(* Logix 5000 AddOnInstructionDefinition export YAI_Assy_155_115_EIP_Hz; software revision 21.03 *)

ADD_ON_INSTRUCTION YAI_Assy_155_115_EIP_Hz   (* revision 1.0, vendor Yaskawa America, Inc. *)
// YAI Assembly 155 and 115
// Help:
// This add-on instruction is for use with input assemblie 166 and output assemblies 116.
// Node_Input_Assy is defined as the node's input assembly integer array.
// Node_Output_Assy is defined as the node's output assembly integer array.
// Torque limit/reference, torque compensation and torque output variables are only available with A1000.
VAR_IN_OUT
   Node_Input_Assy : AB:ETHERNET_MODULE_INT_40Bytes:I:0; {required}   // Input assembly words
   Node_Output_Assy : AB:ETHERNET_MODULE_INT_40Bytes:O:0; {required}   // Output assembly words
END_VAR
VAR_INPUT
   RunFwd : BOOL; {visible}   // Forward run command
   RunRev : BOOL; {visible}   // Reverse run command
   MFI_3 : BOOL; {visible}   // Multi-function input 3
   MFI_4 : BOOL; {visible}   // Multi-function input 4
   MFI_5 : BOOL; {visible}   // Multi-function input 5
   MFI_6 : BOOL; {visible}   // Multi-function input 6
   MFI_7 : BOOL; {visible}   // Multi-function input 7
   MFI_8 : BOOL; {visible}   // Multi-function input 8
   External_Fault : BOOL;   // External fault command (EF0)
   FaultReset : BOOL; {visible}   // Fault reset command
   MFO_1 : BOOL; {visible}   // Multi-function output (M1-M2 for A/P1000, MA/MB/MC for V1000)
   MFO_2 : BOOL; {visible}   // Multi-function output (M3-M4 for A/P1000, P1 for V1000)
   MFO_3 : BOOL; {visible}   // Multi-function output (M5-M6 for A/P1000, P2 for V1000)
   Freq_Ref : REAL; {visible}   // Frequency reference command in Hz (xx.xx resolution)
   Torq_Ref_Limit : REAL; {visible}   // Torque reference/limit (A1000 only)
   Torq_Comp : REAL; {visible}   // Torque compensation command (A1000 only)
   Analog_Output_1 : REAL;   // Analog output 1 level command
   Analog_Output_2 : REAL;   // Analog output 2 level command
   Digital_Output_1 : BOOL;   // Digital output 1 activation - M1-M2
   Digital_Output_2 : BOOL;   // Digital output 2 activation - M3-M4
   Digital_Output_3 : BOOL;   // Digital output 3 activation - M5-M6
   Digital_Output_Fault_Enable : BOOL;   // Bit to enable control of fault output relay over the network
   Digital_Output_Fault : BOOL;   // Fault relay activation - MA-MB-MC
END_VAR
VAR_OUTPUT
   Running : BOOL; {access Read Only, visible}   // Drive running forward status bit
   ZSP : BOOL; {access Read Only, visible}   // Drive zero speed status bit
   RunningRev : BOOL; {access Read Only, visible}   // Drive running reverse status bit
   Reset : BOOL; {access Read Only, visible}   // Drive reset command status bit
   At_Speed : BOOL; {access Read Only, visible}   // Drive at commanded speed status bit
   Ready : BOOL; {access Read Only, visible}   // Drive ready status bit
   Alarm : BOOL; {access Read Only, visible}   // Drive alarm status bit
   Faulted : BOOL; {access Read Only, visible}   // Drive faulted status bit
   OPE : BOOL; {access Read Only}   // OPE alarm/fault present
   UV : BOOL; {access Read Only}   // Drive in UV (undervoltage) state status bit
   NetCtrlStatus : BOOL; {access Read Only, visible}   // Drive network run source status bit (1 = source coming from network)
   MFO_1_Status : BOOL; {access Read Only, visible}   // Drive multi-function output 1 (M1-M2 for A/P1000, MA/MB/MC for V1000) status
   MFO_2_Status : BOOL; {access Read Only, visible}   // Drive multi-function output 1 (M3-M4 for A/P1000, P1 for V1000) status
   MFO_3_Status : BOOL; {access Read Only, visible}   // Drive multi-function output 1 (M5-M6 for A/P1000, P2 for V1000) status
   ZSV : BOOL; {access Read Only, visible}   // Drive zero servo completed status bit
   Motor_Speed : REAL; {access Read Only, visible}   // Motor speed in Hz (xx.xx resolution)
   Torque_Actual : REAL; {access Read Only, visible}   // Drive torque output in % (xxx.x resolution)
   PG1_Count : INT; {access Read Only}   // Encoder feedback count
   Freq_Cmd : REAL; {access Read Only, visible}   // Commanded frequency in Hz (xx.xx resolution)
   Output_Freq : REAL; {access Read Only, visible}   // Drive output frequency in Hz (xx.xx resolution)
   Output_Current : REAL; {access Read Only, visible}   // Drive output current in A (xxx.x resolution)
   Analog_Input_1_Level : REAL; {access Read Only}   // Analog input 1 level in % (xxx.x resolution)
   DC_Bus_Volt : INT; {access Read Only, visible}   // DC bus voltage in Vdc (xxx resolution)
   Analog_Input_3_Level : REAL; {access Read Only}   // Analog input 3 level in % (xxx.x resolution)
   Analog_Input_2_Level : REAL; {access Read Only}   // Analog input 2 level in % (xxx.x resolution)
   S1_Status : BOOL; {access Read Only}   // Digital input S1 status
   S2_Status : BOOL; {access Read Only}   // Digital input S2 status
   S3_Status : BOOL; {access Read Only}   // Digital input S3 status
   S4_Status : BOOL; {access Read Only}   // Digital input S4 status
   S5_Status : BOOL; {access Read Only}   // Digital input S5 status
   S6_Status : BOOL; {access Read Only}   // Digital input S6 status
   S7_Status : BOOL; {access Read Only}   // Digital input S7 status
   S8_Status : BOOL; {access Read Only}   // Digital input S8 status
   PG2_Count : INT;   // Encoder 2 feedback count
   UV_Alarm : BOOL; {access Read Only}   // Undervoltage alarm
   OV_Alarm : BOOL; {access Read Only}   // Overvoltage alarm
   OH_Alarm : BOOL; {access Read Only}   // Overheat alarm
   OH2_Alarm : BOOL; {access Read Only}   // Drive overheat alarm
   OL3_Alarm : BOOL; {access Read Only}   // Overtorque detection 1 alarm
   OL4_Alarm : BOOL; {access Read Only}   // Overtorque detection 2 alarm
   EF_Alarm : BOOL; {access Read Only}   // Run command error alarm
   bb_Alarm : BOOL; {access Read Only}   // Baseblock alarm
   EF3_Alarm : BOOL; {access Read Only}   // External fault 3 alarm
   EF4_Alarm : BOOL; {access Read Only}   // External fault 4 alarm
   EF5_Alarm : BOOL; {access Read Only}   // External fault 5 alarm
   EF6_Alarm : BOOL; {access Read Only}   // External fault 6 alarm
   EF7_Alarm : BOOL; {access Read Only}   // External fault 7 alarm
   EF8_Alarm : BOOL; {access Read Only}   // External fault 8 alarm
   FAN_Alarm : BOOL; {access Read Only}   // Cooling fan error alarm
   OS_Alarm : BOOL; {access Read Only}   // Overspeed alarm
   DEV_Alarm : BOOL; {access Read Only}   // Speed deviation alarm
   PGO_Alarm : BOOL; {access Read Only}   // Encoder feedback open alarm
   OPR_Alarm : BOOL; {access Read Only}   // Operator removed alarm
   CE_Alarm : BOOL; {access Read Only}   // Serial communication error alarm
   BUS_Alarm : BOOL; {access Read Only}   // BUS alarm
   CALL_Alarm : BOOL; {access Read Only}   // Serial communication timeout alarm
   OL1_Alarm : BOOL; {access Read Only}   // Motor overload alarm
   OL2_Alarm : BOOL; {access Read Only}   // Drive overload alarm
   EF0_Alarm : BOOL; {access Read Only}   // External fault 0 alarm
   RUN_Alarm : BOOL; {access Read Only}   // Motor 2 run command issued while running alarm
   UL3_Alarm : BOOL; {access Read Only}   // Undertorque detecxtion 1 alarm
   UL4_Alarm : BOOL; {access Read Only}   // Undertorque detection 2 alarm
   SE_Alarm : BOOL; {access Read Only}   // Modbus test failure alarm
   OH3_Alarm : BOOL; {access Read Only}   // Motor overload alarm
   FBL_Alarm : BOOL; {access Read Only}   // PID feedback loss alarm
   FBH_Alarm : BOOL; {access Read Only}   // PID feedback loss alarm
   DNE_Alarm : BOOL; {access Read Only}   // Drive not enabled alarm
END_VAR
VAR
   FRef_Convert : DINT;
   FOut_Convert : REAL;
   FOut_Temp : REAL;
   TRef_Convert : INT;
   TComp_Convert : INT;
   TOut_Convert : REAL;
   TOut_Temp : REAL;
   IOut_Temp : REAL;
   IOut_Convert : REAL;
   AO1_Convert : INT;
   AO2_Convert : INT;
   Motor_Speed_Temp : REAL;
   Motor_Speed_Convert : REAL;
   Freq_Cmd_Temp : REAL;
   Freq_Cmd_Convert : REAL;
   AI1_Temp : REAL;
   AI1_Convert : REAL;
   AI2_Temp : REAL; {access None}
   AI2_Convert : REAL; {access None}
   AI3_Temp : REAL; {access None}
   AI3_Convert : REAL; {access None}
END_VAR

ROUTINE Logic   (* ladder *)
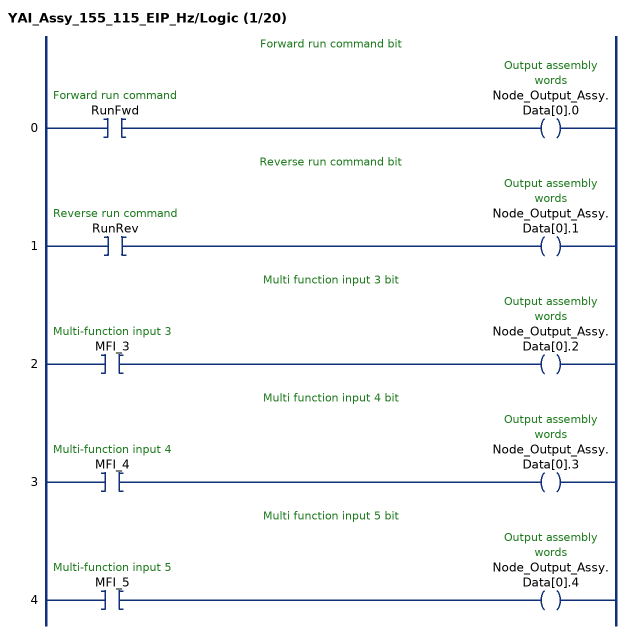
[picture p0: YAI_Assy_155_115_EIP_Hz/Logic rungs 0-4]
   // Forward run command bit
   0: XIC(RunFwd)OTE(Node_Output_Assy.Data[0].0);
   // Reverse run command bit
   1: XIC(RunRev)OTE(Node_Output_Assy.Data[0].1);
   // Multi function input 3 bit
   2: XIC(MFI_3)OTE(Node_Output_Assy.Data[0].2);
   // Multi function input 4 bit
   3: XIC(MFI_4)OTE(Node_Output_Assy.Data[0].3);
   // Multi function input 5 bit
   4: XIC(MFI_5)OTE(Node_Output_Assy.Data[0].4);
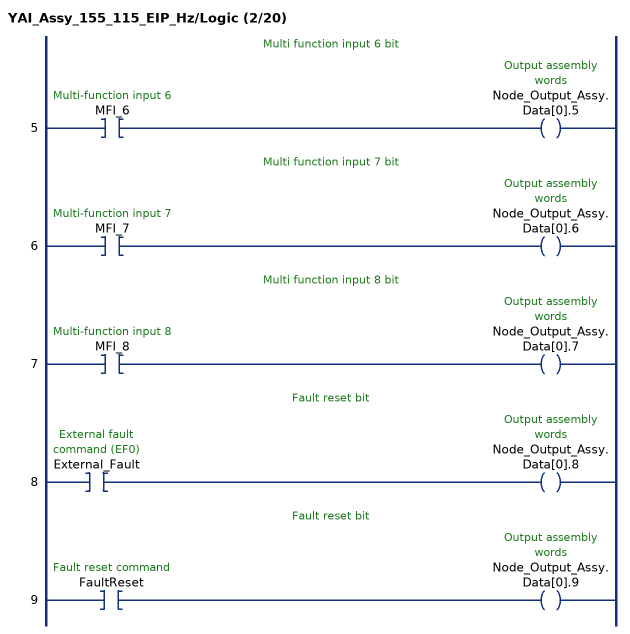
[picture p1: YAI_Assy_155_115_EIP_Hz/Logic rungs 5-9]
   // Multi function input 6 bit
   5: XIC(MFI_6)OTE(Node_Output_Assy.Data[0].5);
   // Multi function input 7 bit
   6: XIC(MFI_7)OTE(Node_Output_Assy.Data[0].6);
   // Multi function input 8 bit
   7: XIC(MFI_8)OTE(Node_Output_Assy.Data[0].7);
   // Fault reset bit
   8: XIC(External_Fault)OTE(Node_Output_Assy.Data[0].8);
   // Fault reset bit
   9: XIC(FaultReset)OTE(Node_Output_Assy.Data[0].9);
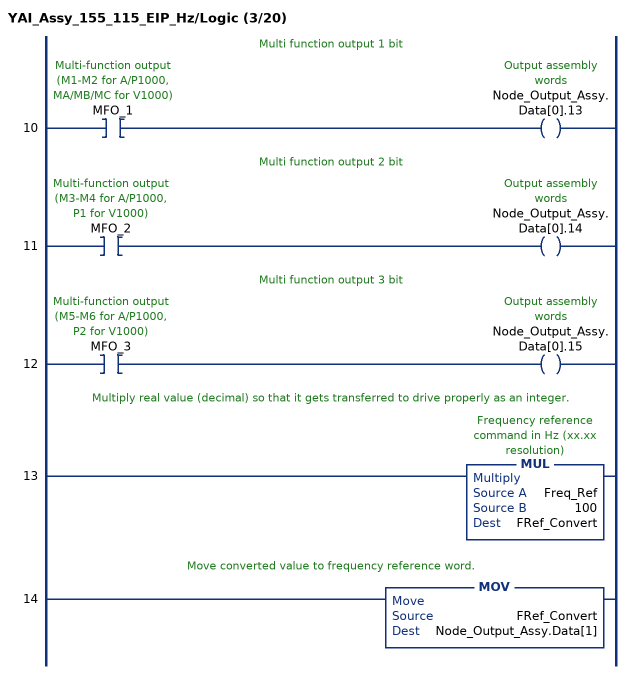
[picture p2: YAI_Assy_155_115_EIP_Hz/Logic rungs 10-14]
   // Multi function output 1 bit
   10: XIC(MFO_1)OTE(Node_Output_Assy.Data[0].13);
   // Multi function output 2 bit
   11: XIC(MFO_2)OTE(Node_Output_Assy.Data[0].14);
   // Multi function output 3 bit
   12: XIC(MFO_3)OTE(Node_Output_Assy.Data[0].15);
   // Multiply real value (decimal) so that it gets transferred to drive properly as an integer.
   13: MUL(Freq_Ref,100,FRef_Convert);
   // Move converted value to frequency reference word.
   14: MOV(FRef_Convert,Node_Output_Assy.Data[1]);
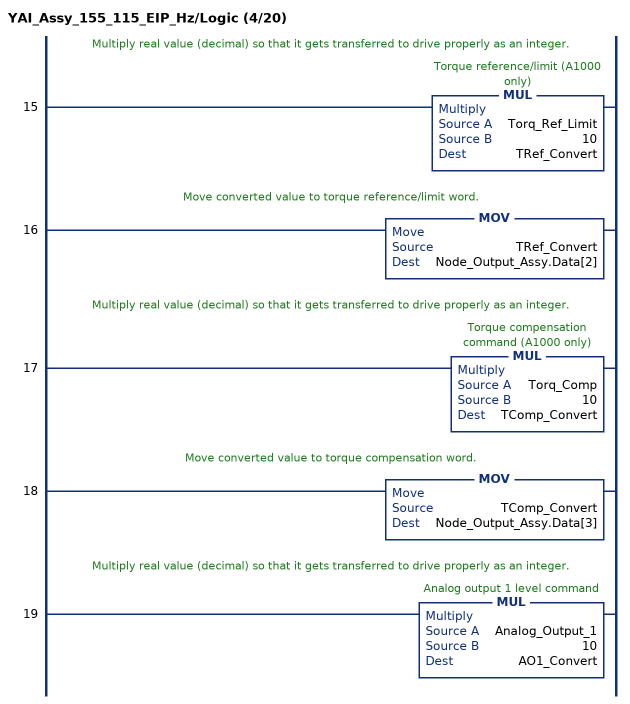
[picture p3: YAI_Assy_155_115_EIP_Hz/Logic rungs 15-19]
   // Multiply real value (decimal) so that it gets transferred to drive properly as an integer.
   15: MUL(Torq_Ref_Limit,10,TRef_Convert);
   // Move converted value to torque reference/limit word.
   16: MOV(TRef_Convert,Node_Output_Assy.Data[2]);
   // Multiply real value (decimal) so that it gets transferred to drive properly as an integer.
   17: MUL(Torq_Comp,10,TComp_Convert);
   // Move converted value to torque compensation word.
   18: MOV(TComp_Convert,Node_Output_Assy.Data[3]);
   // Multiply real value (decimal) so that it gets transferred to drive properly as an integer.
   19: MUL(Analog_Output_1,10,AO1_Convert);
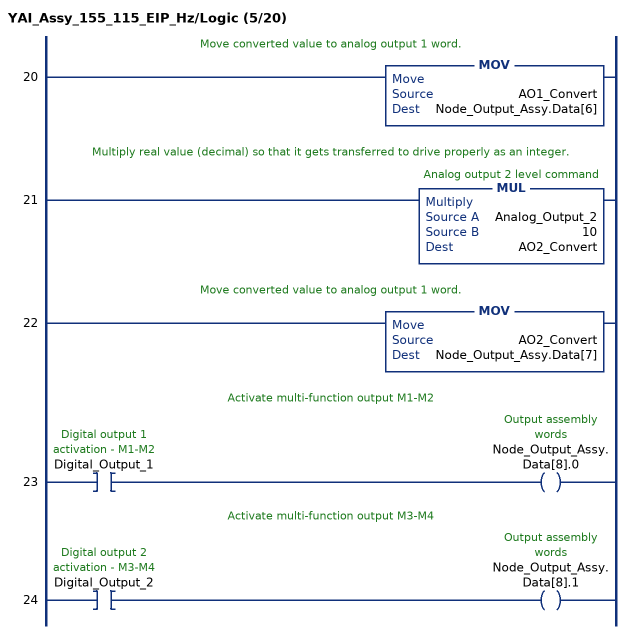
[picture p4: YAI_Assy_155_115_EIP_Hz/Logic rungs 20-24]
   // Move converted value to analog output 1 word.
   20: MOV(AO1_Convert,Node_Output_Assy.Data[6]);
   // Multiply real value (decimal) so that it gets transferred to drive properly as an integer.
   21: MUL(Analog_Output_2,10,AO2_Convert);
   // Move converted value to analog output 1 word.
   22: MOV(AO2_Convert,Node_Output_Assy.Data[7]);
   // Activate multi-function output M1-M2
   23: XIC(Digital_Output_1)OTE(Node_Output_Assy.Data[8].0);
   // Activate multi-function output M3-M4
   24: XIC(Digital_Output_2)OTE(Node_Output_Assy.Data[8].1);
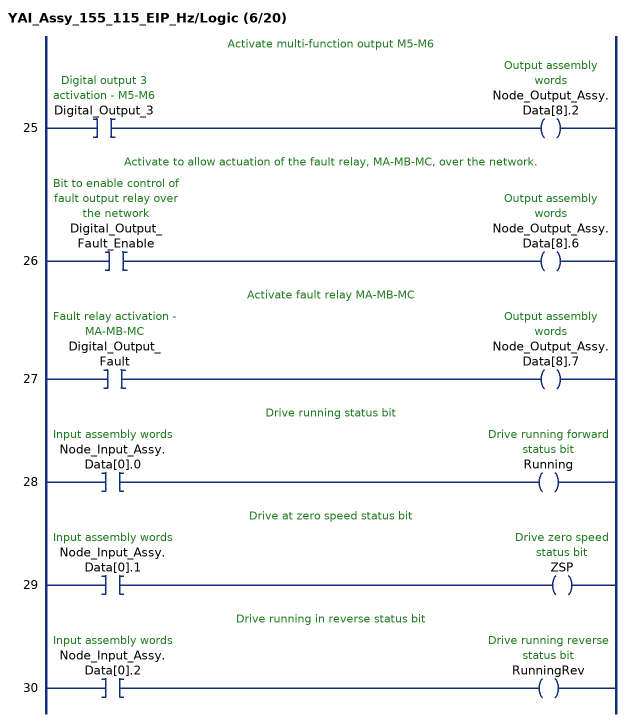
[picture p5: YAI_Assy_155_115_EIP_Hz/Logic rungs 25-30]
   // Activate multi-function output M5-M6
   25: XIC(Digital_Output_3)OTE(Node_Output_Assy.Data[8].2);
   // Activate to allow actuation of the fault relay, MA-MB-MC, over the network.
   26: XIC(Digital_Output_Fault_Enable)OTE(Node_Output_Assy.Data[8].6);
   // Activate fault relay MA-MB-MC
   27: XIC(Digital_Output_Fault)OTE(Node_Output_Assy.Data[8].7);
   // Drive running status bit
   28: XIC(Node_Input_Assy.Data[0].0)OTE(Running);
   // Drive at zero speed status bit
   29: XIC(Node_Input_Assy.Data[0].1)OTE(ZSP);
   // Drive running in reverse status bit
   30: XIC(Node_Input_Assy.Data[0].2)OTE(RunningRev);
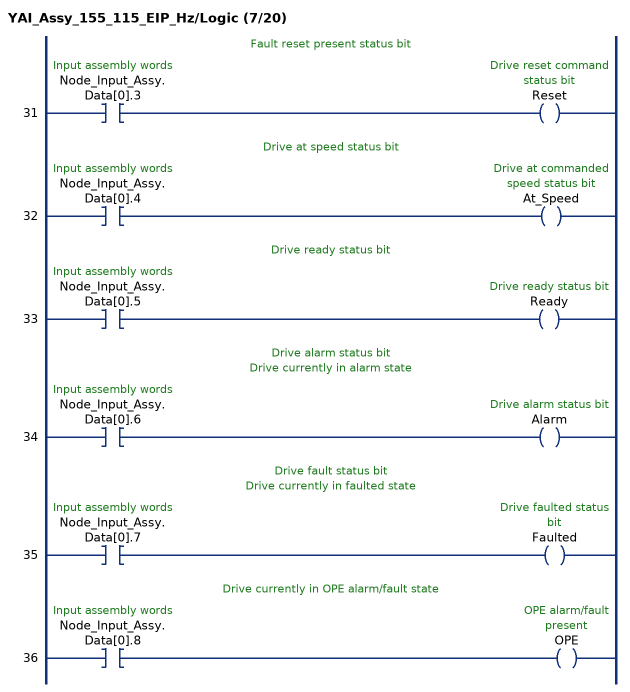
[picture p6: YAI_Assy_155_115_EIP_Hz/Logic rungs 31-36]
   // Fault reset present status bit
   31: XIC(Node_Input_Assy.Data[0].3)OTE(Reset);
   // Drive at speed status bit
   32: XIC(Node_Input_Assy.Data[0].4)OTE(At_Speed);
   // Drive ready status bit
   33: XIC(Node_Input_Assy.Data[0].5)OTE(Ready);
   // Drive alarm status bit
   // Drive currently in alarm state
   34: XIC(Node_Input_Assy.Data[0].6)OTE(Alarm);
   // Drive fault status bit
   // Drive currently in faulted state
   35: XIC(Node_Input_Assy.Data[0].7)OTE(Faulted);
   // Drive currently in OPE alarm/fault state
   36: XIC(Node_Input_Assy.Data[0].8)OTE(OPE);
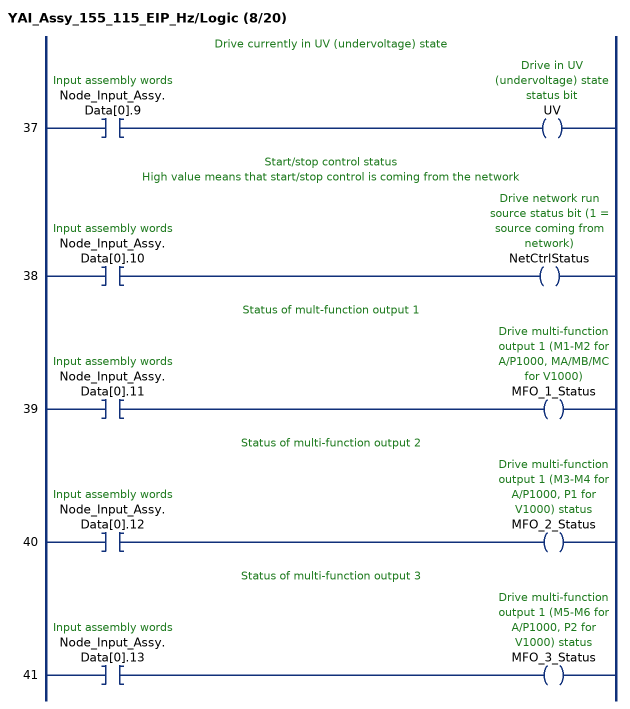
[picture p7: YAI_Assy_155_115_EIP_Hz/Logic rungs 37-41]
   // Drive currently in UV (undervoltage) state
   37: XIC(Node_Input_Assy.Data[0].9)OTE(UV);
   // Start/stop control status
   // High value means that start/stop control is coming from the network
   38: XIC(Node_Input_Assy.Data[0].10)OTE(NetCtrlStatus);
   // Status of mult-function output 1
   39: XIC(Node_Input_Assy.Data[0].11)OTE(MFO_1_Status);
   // Status of multi-function output 2
   40: XIC(Node_Input_Assy.Data[0].12)OTE(MFO_2_Status);
   // Status of multi-function output 3
   41: XIC(Node_Input_Assy.Data[0].13)OTE(MFO_3_Status);
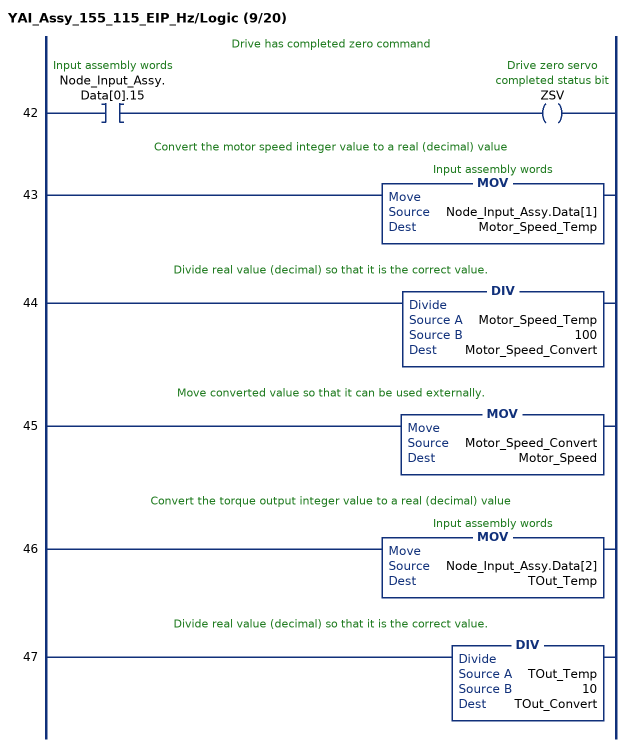
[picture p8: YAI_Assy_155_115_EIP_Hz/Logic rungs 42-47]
   // Drive has completed zero command
   42: XIC(Node_Input_Assy.Data[0].15)OTE(ZSV);
   // Convert the motor speed integer value to a real (decimal) value
   43: MOV(Node_Input_Assy.Data[1],Motor_Speed_Temp);
   // Divide real value (decimal) so that it is the correct value.
   44: DIV(Motor_Speed_Temp,100,Motor_Speed_Convert);
   // Move converted value so that it can be used externally.
   45: MOV(Motor_Speed_Convert,Motor_Speed);
   // Convert the torque output integer value to a real (decimal) value
   46: MOV(Node_Input_Assy.Data[2],TOut_Temp);
   // Divide real value (decimal) so that it is the correct value.
   47: DIV(TOut_Temp,10,TOut_Convert);
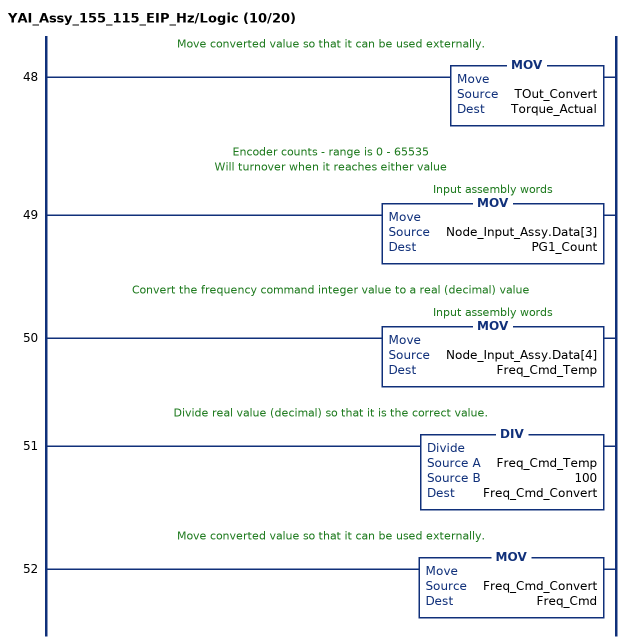
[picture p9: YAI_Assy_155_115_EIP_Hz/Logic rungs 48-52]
   // Move converted value so that it can be used externally.
   48: MOV(TOut_Convert,Torque_Actual);
   // Encoder counts - range is 0 - 65535
   // Will turnover when it reaches either value
   49: MOV(Node_Input_Assy.Data[3],PG1_Count);
   // Convert the frequency command integer value to a real (decimal) value
   50: MOV(Node_Input_Assy.Data[4],Freq_Cmd_Temp);
   // Divide real value (decimal) so that it is the correct value.
   51: DIV(Freq_Cmd_Temp,100,Freq_Cmd_Convert);
   // Move converted value so that it can be used externally.
   52: MOV(Freq_Cmd_Convert,Freq_Cmd);
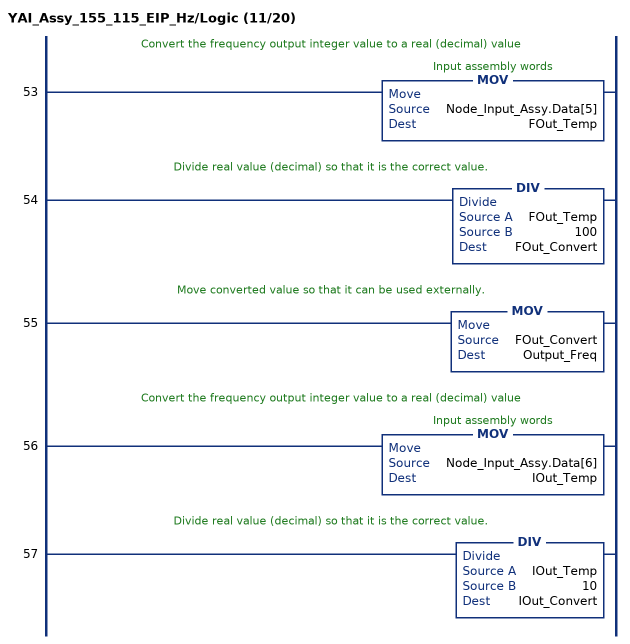
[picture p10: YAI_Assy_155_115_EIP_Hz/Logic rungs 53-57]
   // Convert the frequency output integer value to a real (decimal) value
   53: MOV(Node_Input_Assy.Data[5],FOut_Temp);
   // Divide real value (decimal) so that it is the correct value.
   54: DIV(FOut_Temp,100,FOut_Convert);
   // Move converted value so that it can be used externally.
   55: MOV(FOut_Convert,Output_Freq);
   // Convert the frequency output integer value to a real (decimal) value
   56: MOV(Node_Input_Assy.Data[6],IOut_Temp);
   // Divide real value (decimal) so that it is the correct value.
   57: DIV(IOut_Temp,10,IOut_Convert);
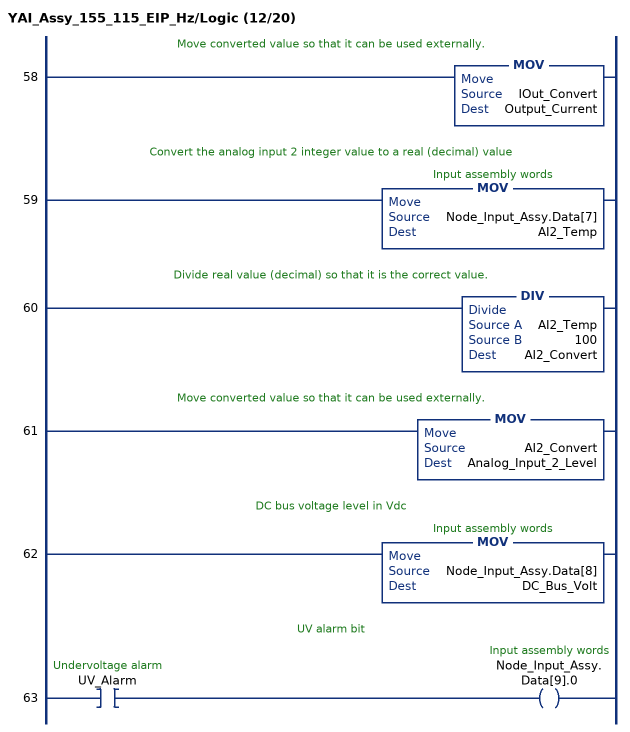
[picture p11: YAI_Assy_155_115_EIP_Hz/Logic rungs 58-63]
   // Move converted value so that it can be used externally.
   58: MOV(IOut_Convert,Output_Current);
   // Convert the analog input 2 integer value to a real (decimal) value
   59: MOV(Node_Input_Assy.Data[7],AI2_Temp);
   // Divide real value (decimal) so that it is the correct value.
   60: DIV(AI2_Temp,100,AI2_Convert);
   // Move converted value so that it can be used externally.
   61: MOV(AI2_Convert,Analog_Input_2_Level);
   // DC bus voltage level in Vdc
   62: MOV(Node_Input_Assy.Data[8],DC_Bus_Volt);
   // UV alarm bit
   63: XIC(UV_Alarm)OTE(Node_Input_Assy.Data[9].0);
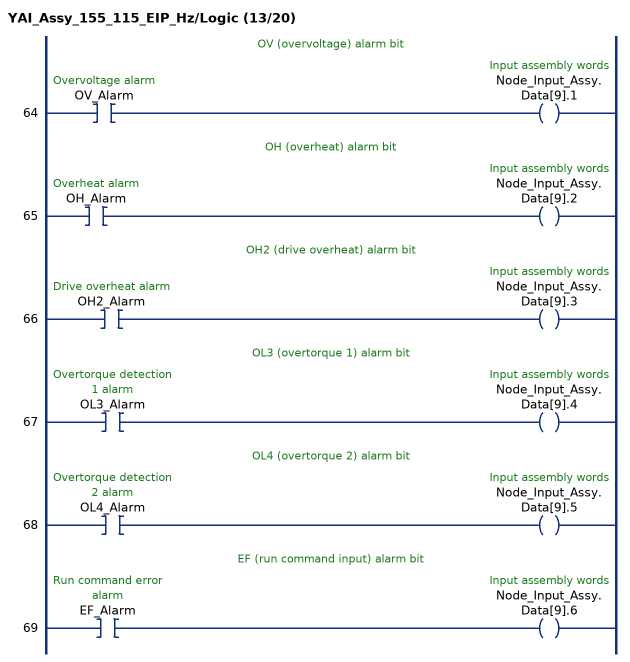
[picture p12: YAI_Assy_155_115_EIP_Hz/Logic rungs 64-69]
   // OV (overvoltage) alarm bit
   64: XIC(OV_Alarm)OTE(Node_Input_Assy.Data[9].1);
   // OH (overheat) alarm bit
   65: XIC(OH_Alarm)OTE(Node_Input_Assy.Data[9].2);
   // OH2 (drive overheat) alarm bit
   66: XIC(OH2_Alarm)OTE(Node_Input_Assy.Data[9].3);
   // OL3 (overtorque 1) alarm bit
   67: XIC(OL3_Alarm)OTE(Node_Input_Assy.Data[9].4);
   // OL4 (overtorque 2) alarm bit
   68: XIC(OL4_Alarm)OTE(Node_Input_Assy.Data[9].5);
   // EF (run command input) alarm bit
   69: XIC(EF_Alarm)OTE(Node_Input_Assy.Data[9].6);
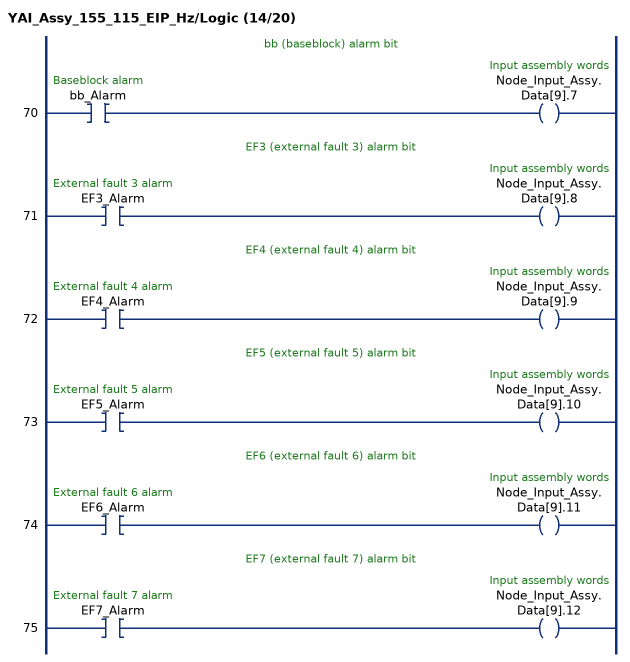
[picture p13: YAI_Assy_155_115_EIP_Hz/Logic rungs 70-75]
   // bb (baseblock) alarm bit
   70: XIC(bb_Alarm)OTE(Node_Input_Assy.Data[9].7);
   // EF3 (external fault 3) alarm bit
   71: XIC(EF3_Alarm)OTE(Node_Input_Assy.Data[9].8);
   // EF4 (external fault 4) alarm bit
   72: XIC(EF4_Alarm)OTE(Node_Input_Assy.Data[9].9);
   // EF5 (external fault 5) alarm bit
   73: XIC(EF5_Alarm)OTE(Node_Input_Assy.Data[9].10);
   // EF6 (external fault 6) alarm bit
   74: XIC(EF6_Alarm)OTE(Node_Input_Assy.Data[9].11);
   // EF7 (external fault 7) alarm bit
   75: XIC(EF7_Alarm)OTE(Node_Input_Assy.Data[9].12);
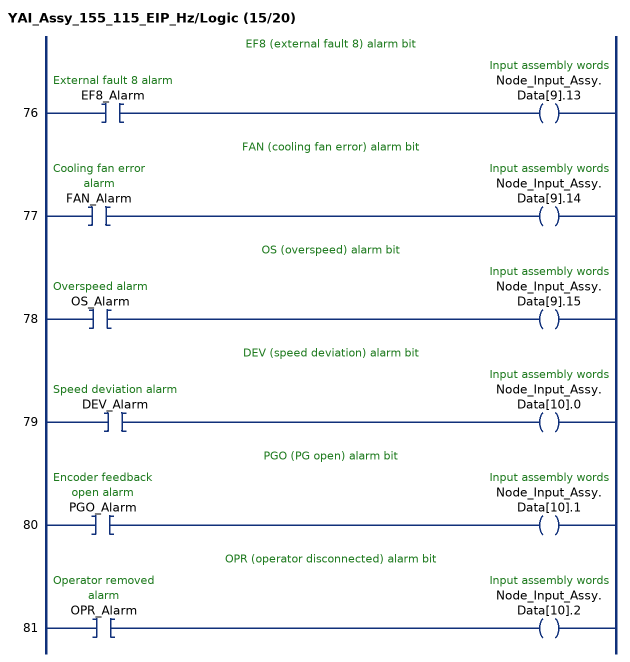
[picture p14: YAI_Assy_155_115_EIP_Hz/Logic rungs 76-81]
   // EF8 (external fault 8) alarm bit
   76: XIC(EF8_Alarm)OTE(Node_Input_Assy.Data[9].13);
   // FAN (cooling fan error) alarm bit
   77: XIC(FAN_Alarm)OTE(Node_Input_Assy.Data[9].14);
   // OS (overspeed) alarm bit
   78: XIC(OS_Alarm)OTE(Node_Input_Assy.Data[9].15);
   // DEV (speed deviation) alarm bit
   79: XIC(DEV_Alarm)OTE(Node_Input_Assy.Data[10].0);
   // PGO (PG open) alarm bit
   80: XIC(PGO_Alarm)OTE(Node_Input_Assy.Data[10].1);
   // OPR (operator disconnected) alarm bit
   81: XIC(OPR_Alarm)OTE(Node_Input_Assy.Data[10].2);
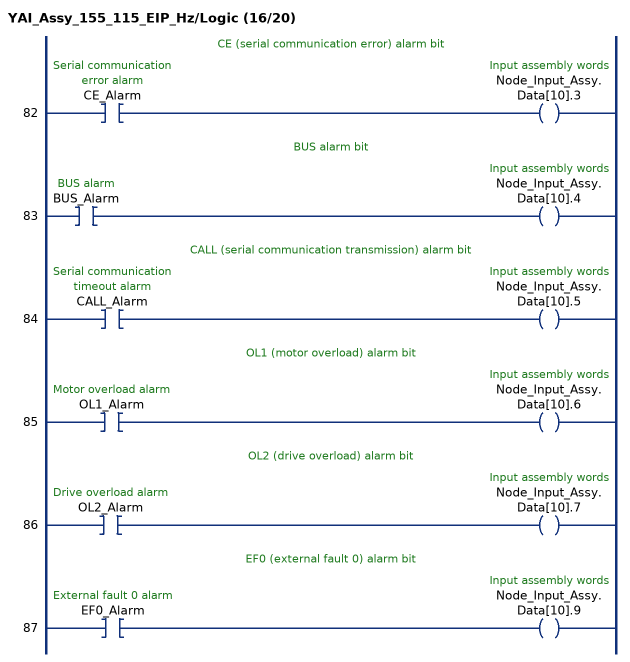
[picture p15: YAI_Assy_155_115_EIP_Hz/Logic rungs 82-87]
   // CE (serial communication error) alarm bit
   82: XIC(CE_Alarm)OTE(Node_Input_Assy.Data[10].3);
   // BUS alarm bit
   83: XIC(BUS_Alarm)OTE(Node_Input_Assy.Data[10].4);
   // CALL (serial communication transmission) alarm bit
   84: XIC(CALL_Alarm)OTE(Node_Input_Assy.Data[10].5);
   // OL1 (motor overload) alarm bit
   85: XIC(OL1_Alarm)OTE(Node_Input_Assy.Data[10].6);
   // OL2 (drive overload) alarm bit
   86: XIC(OL2_Alarm)OTE(Node_Input_Assy.Data[10].7);
   // EF0 (external fault 0) alarm bit
   87: XIC(EF0_Alarm)OTE(Node_Input_Assy.Data[10].9);
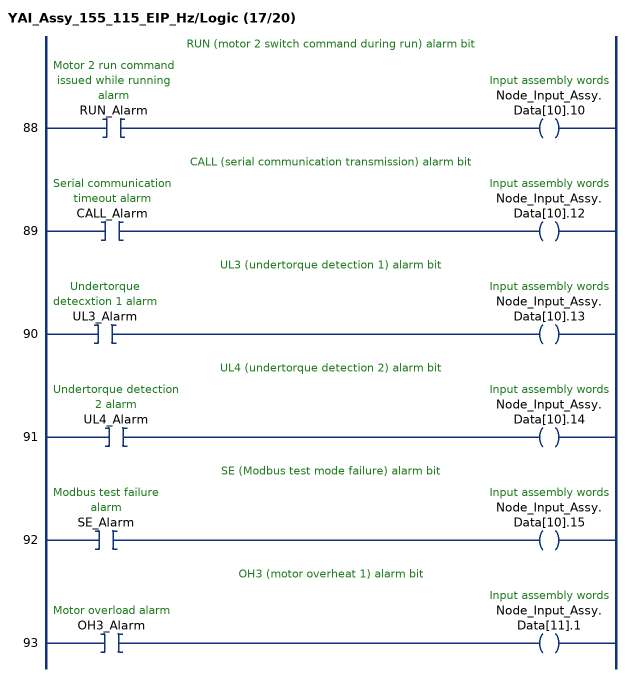
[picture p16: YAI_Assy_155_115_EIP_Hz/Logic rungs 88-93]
   // RUN (motor 2 switch command during run) alarm bit
   88: XIC(RUN_Alarm)OTE(Node_Input_Assy.Data[10].10);
   // CALL (serial communication transmission) alarm bit
   89: XIC(CALL_Alarm)OTE(Node_Input_Assy.Data[10].12);
   // UL3 (undertorque detection 1) alarm bit
   90: XIC(UL3_Alarm)OTE(Node_Input_Assy.Data[10].13);
   // UL4 (undertorque detection 2) alarm bit
   91: XIC(UL4_Alarm)OTE(Node_Input_Assy.Data[10].14);
   // SE (Modbus test mode failure) alarm bit
   92: XIC(SE_Alarm)OTE(Node_Input_Assy.Data[10].15);
   // OH3 (motor overheat 1) alarm bit
   93: XIC(OH3_Alarm)OTE(Node_Input_Assy.Data[11].1);
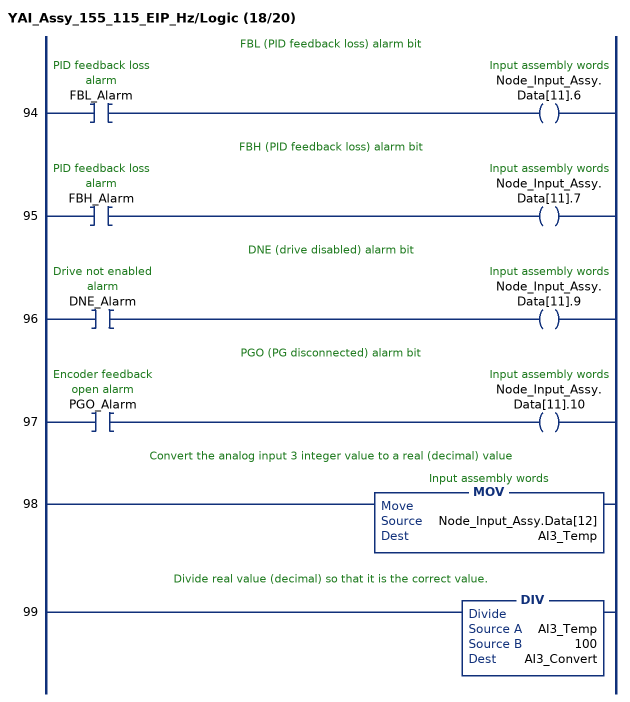
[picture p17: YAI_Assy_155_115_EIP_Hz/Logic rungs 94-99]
   // FBL (PID feedback loss) alarm bit
   94: XIC(FBL_Alarm)OTE(Node_Input_Assy.Data[11].6);
   // FBH (PID feedback loss) alarm bit
   95: XIC(FBH_Alarm)OTE(Node_Input_Assy.Data[11].7);
   // DNE (drive disabled) alarm bit
   96: XIC(DNE_Alarm)OTE(Node_Input_Assy.Data[11].9);
   // PGO (PG disconnected) alarm bit
   97: XIC(PGO_Alarm)OTE(Node_Input_Assy.Data[11].10);
   // Convert the analog input 3 integer value to a real (decimal) value
   98: MOV(Node_Input_Assy.Data[12],AI3_Temp);
   // Divide real value (decimal) so that it is the correct value.
   99: DIV(AI3_Temp,100,AI3_Convert);
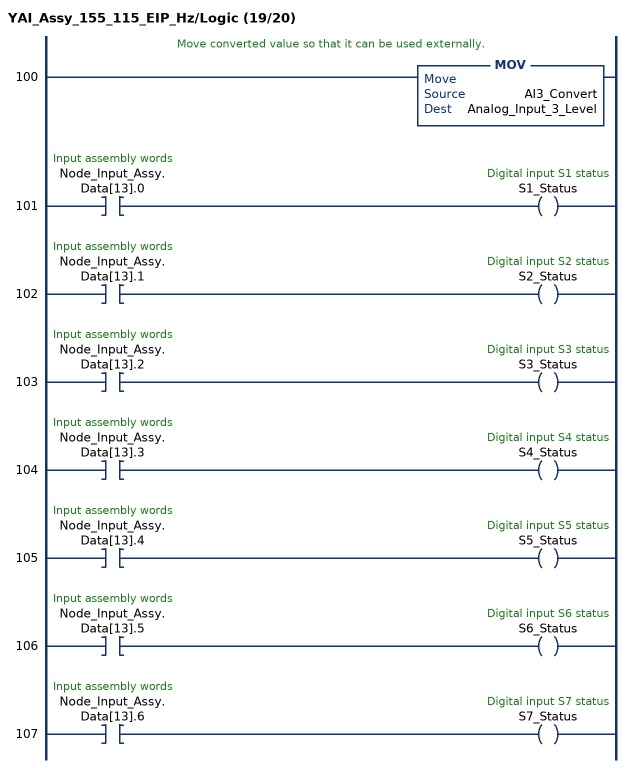
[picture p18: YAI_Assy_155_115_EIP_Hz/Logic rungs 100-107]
   // Move converted value so that it can be used externally.
   100: MOV(AI3_Convert,Analog_Input_3_Level);
   101: XIC(Node_Input_Assy.Data[13].0)OTE(S1_Status);
   102: XIC(Node_Input_Assy.Data[13].1)OTE(S2_Status);
   103: XIC(Node_Input_Assy.Data[13].2)OTE(S3_Status);
   104: XIC(Node_Input_Assy.Data[13].3)OTE(S4_Status);
   105: XIC(Node_Input_Assy.Data[13].4)OTE(S5_Status);
   106: XIC(Node_Input_Assy.Data[13].5)OTE(S6_Status);
   107: XIC(Node_Input_Assy.Data[13].6)OTE(S7_Status);
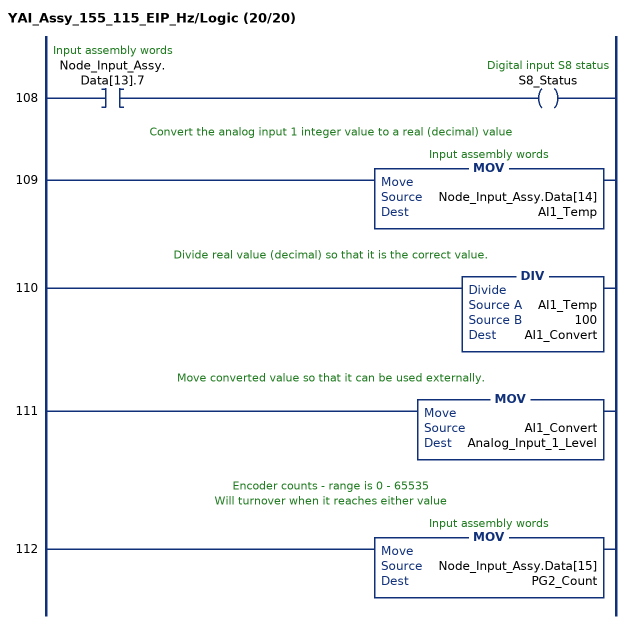
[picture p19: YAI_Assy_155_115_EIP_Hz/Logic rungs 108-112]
   108: XIC(Node_Input_Assy.Data[13].7)OTE(S8_Status);
   // Convert the analog input 1 integer value to a real (decimal) value
   109: MOV(Node_Input_Assy.Data[14],AI1_Temp);
   // Divide real value (decimal) so that it is the correct value.
   110: DIV(AI1_Temp,100,AI1_Convert);
   // Move converted value so that it can be used externally.
   111: MOV(AI1_Convert,Analog_Input_1_Level);
   // Encoder counts - range is 0 - 65535
   // Will turnover when it reaches either value
   112: MOV(Node_Input_Assy.Data[15],PG2_Count);
END_ROUTINE
END_ADD_ON_INSTRUCTION
